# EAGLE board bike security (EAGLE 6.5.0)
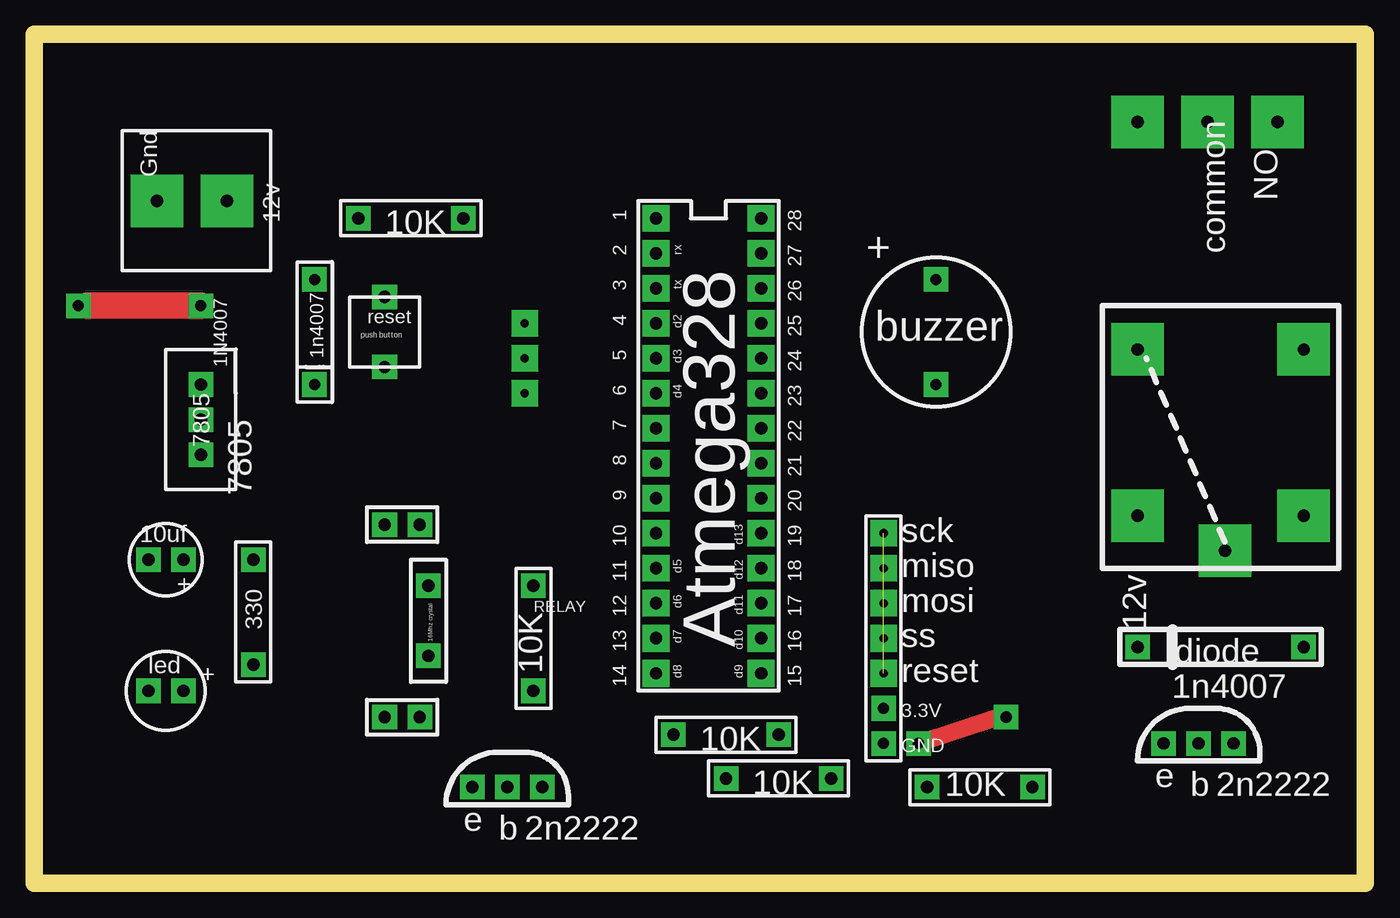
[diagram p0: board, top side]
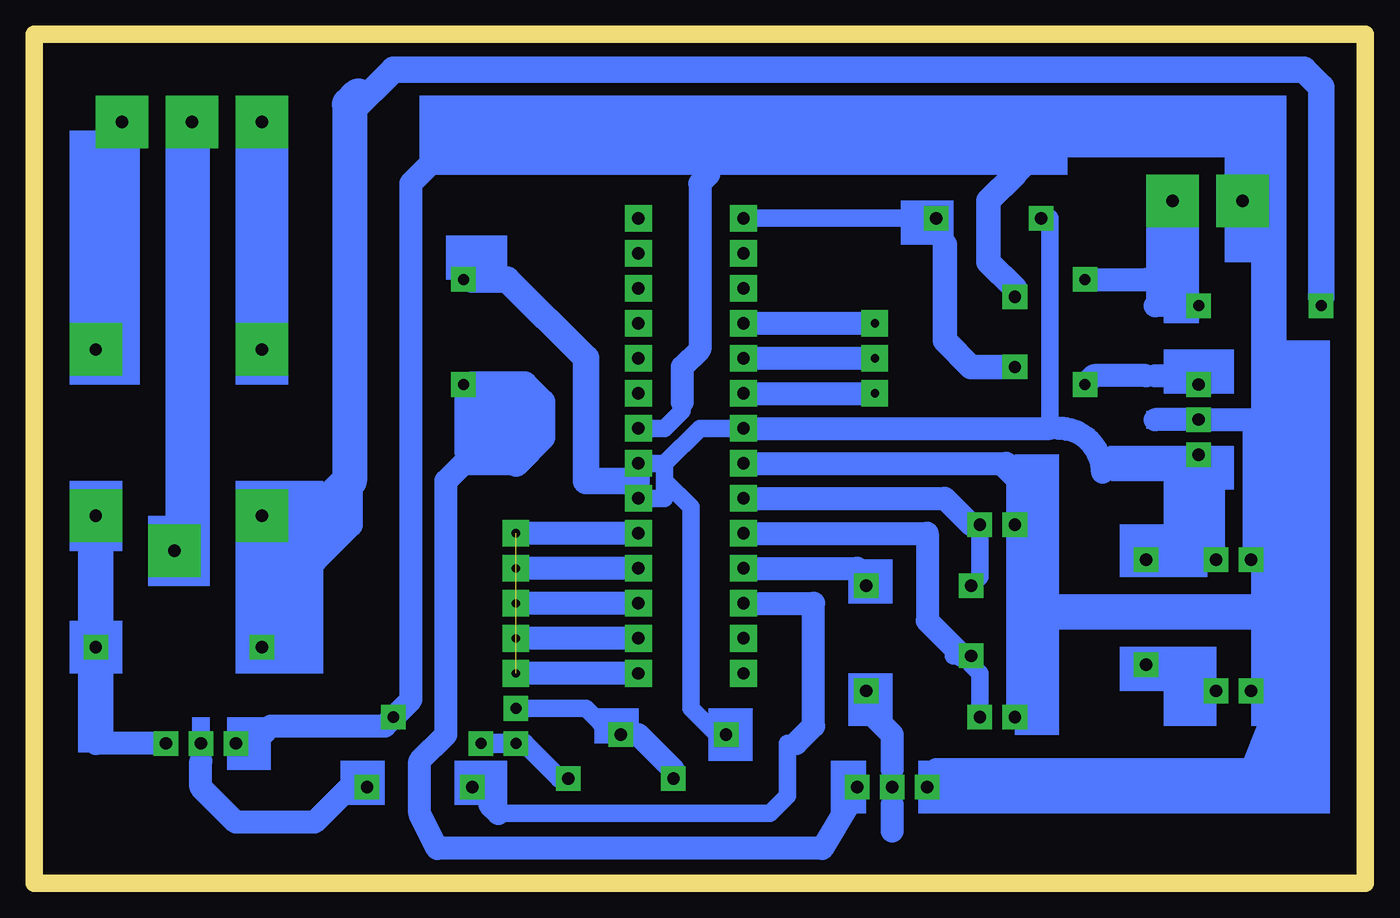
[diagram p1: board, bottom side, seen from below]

Size 96.52 x 61.59 mm. Coordinates in mm from the lower left corner, seen from the top.
Outline: 0,0 96.52,0 96.52,61.59 0,61.59 0,0
Copper layers (1*16): Top 0.035mm / dielectric 1.5mm / Bottom 0.035mm
Design rules "default": minimum track width 10mil, minimum drill 24mil, track to track 8mil, track to pad 8mil, pad to pad 8mil, via to via 8mil, smd to smd 8mil, copper to edge 40mil, drill to drill 8mil, minimum pad ring 10mil, minimum via ring 8mil, stop-mask expansion 4mil, vias tented up to drill 0mil, thermal gap 10mil

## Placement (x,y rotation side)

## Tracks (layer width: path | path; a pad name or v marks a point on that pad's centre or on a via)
S$1
  Bottom 1.27: 29.21,16.51 29.84,16.51 29.84,17.14 31.75,19.05
  Bottom 1.676: 44.45,25.4 31.75,25.4 31.75,19.05 29.21,16.51
S$2  (via drill 0.9 pad 1.93)
  Bottom 1.676: v52.7,27.94 52.7,29.84
  other vias: 52.7,48.26 52.7,45.72 52.7,43.18 52.7,40.64 52.7,38.1 52.7,35.56 52.7,33.02 52.7,30.48 52.7,25.4 52.7,22.86 52.7,20.32 52.7,17.78 45.09,48.26 45.09,45.72 45.09,43.18 45.09,40.64 45.09,38.1 45.09,35.56 45.09,33.02 45.09,30.48 45.09,27.94 45.09,25.4 45.09,22.86 45.09,20.32 45.09,17.78 45.09,15.24
S$3  (via drill 0.8 pad 1.78)
  Bottom 1.676: 80.01,10.79 79.38,11.43 71.12,11.43 v70.48,12.06 69.22,13.34 69.22,50.8 67.31,52.7
S$5  (via drill 0.6 pad 1.93)
  other vias: 35.56,40.64
S$6  (via drill 0.6 pad 1.93)
  other vias: 35.56,38.1
S$7  (via drill 0.9 pad 1.93)
  Bottom 1.27: v52.7,15.24 53.34,15.24
  Bottom 1.676: v52.7,15.24 60.96,15.24 | 52.7,17.78 60.96,17.78 | 52.7,20.32 60.96,20.32 | 52.7,22.86 60.96,22.86 | 52.7,25.4 60.96,25.4
S$8  (via drill 0.6 pad 1.93)
  other vias: 35.56,35.56
S$9  (via drill 0.9 pad 1.78)
  other vias: 80.01,38.73
S$10  (via drill 0.9 pad 1.78)
  other vias: 80.01,26.67
S$11  (via drill 0.9 pad 1.78)
  other vias: 80.01,26.67
S$12  (via drill 0.6 pad 1.93)  (4 unrouted)
  other vias: 61.59,15.24 61.59,17.78 61.59,20.32 61.59,22.86 61.59,25.4
S$13
  Bottom 1.676: 44.45,40.64 36.2,40.64
S$14
  Bottom 1.676: 44.45,38.1 36.2,38.1
S$15
  Bottom 1.676: 44.45,35.56 36.2,35.56
S$16  (via drill 0.9 pad 1.78)
  other vias: 92.08,26.67
S$17  (via drill 0.9 pad 1.78)
  other vias: 80.01,38.73
S$19  (via drill 0.9 pad 1.78)
  other vias: 80.01,38.73
S$20  (via drill 0.9 pad 1.78)
  other vias: 92.08,38.73
S$21  (via drill 0.9 pad 1.78)
  other vias: 86.36,24.13
S$22  (via drill 0.9 pad 1.78)
  other vias: 80.01,17.14
S$23  (via drill 0.9 pad 1.78)
  other vias: 92.08,17.14
S$24
  Bottom 0.813: 80.01,20.95 80.01,19.05
  Bottom 1.422: 80.01,18.41 80.01,20.95
S$25
  Bottom 1.422: 92.08,18.41 92.08,24.77 92.71,24.77
S$26
  Bottom 1.27: 85.72,26.67 85.72,53.98
S$27  (via drill 0.9 pad 3.81)
  other vias: 85.09,55.24 80.01,55.24 80.01,38.73 92.08,38.73 80.01,26.67 86.36,24.13 92.08,26.67
S$28  (via drill 0.9 pad 3.81)
  other vias: 90.17,55.24
S$29
  Bottom 1.27: 92.08,40.64 90.81,41.91 90.81,53.98
S$30
  Bottom 1.676: 87.63,10.16 92.08,10.16
S$31
  Bottom 1.676: 73.66,6.99 76.2,4.45 81.92,4.45 84.45,6.99 84.45,8.89
S$32  (via drill 0.9 pad 1.78)
  other vias: 31.75,6.99
S$33  (via drill 0.9 pad 1.78)
  other vias: 34.29,6.99
S$34  (via drill 0.9 pad 1.78)
  other vias: 36.83,6.99
S$35
  Bottom 1.676: 34.29,8.26 34.29,10.79 35.56,12.06 35.56,12.7
S$36
  Bottom 1.676: 34.29,3.81 34.29,5.71
S$37  (via drill 0.9 pad 1.78)
  other vias: 36.2,21.59
S$38  (via drill 0.9 pad 1.78)
  other vias: 36.2,13.97
S$39
  Bottom 1.676: 6.99,11.43 8.26,8.26 31.11,8.26
S$40
  Bottom 1.676: 6.35,12.06 8.26,6.99 31.11,6.99
S$41
  Bottom 1.676: 37.47,5.71 39.37,2.54 67.31,2.54 68.58,5.08 68.58,8.89 66.67,10.79 66.67,29.21 65.41,30.48 61.59,30.48
  Bottom 1.93: 61.59,30.48 59.69,32.38 59.69,34.92 60.96,36.2 64.77,36.2
S$42  (via drill 0.8 pad 1.78)
  Bottom 1.676: v20.32,43.81 15.88,43.81
S$43
  Bottom 1.676: 19.05,29.84 arc-90 22.23,33.02
S$44
  Bottom 1.676: 13.97,41.91 15.24,41.91
S$45
  Bottom 1.676: 15.24,36.83 13.97,36.83
S$46  (via drill 0.8 pad 1.78)
  other vias: 65.41,43.81
S$47
  Bottom 1.93: 53.34,29.21 56.52,29.21 56.52,38.1 62.23,43.81 64.77,43.81
S$48  (via drill 0.8 pad 1.78)
  Top 1.93: v12.06,41.91 3.81,41.91
S$49  (via drill 0.8 pad 1.78)
  other vias: 65.41,36.2
S$50  (via drill 0.8 pad 1.78)
  other vias: 3.17,41.91
S$51
  Bottom 1.93: 3.17,42.55 3.17,57.78 4.45,59.05 70.48,59.05 73.66,55.88 73.66,29.21 73.66,26.04 76.2,23.5 76.83,23.5
  Bottom 2.54: 73.03,57.15 73.66,56.52 73.66,29.21 74.93,27.94 74.93,25.4
S$52  (via drill 0.9 pad 1.78)
  other vias: 46.35,10.79
S$53  (via drill 0.9 pad 1.78)
  other vias: 53.98,10.79
S$54  (via drill 0.9 pad 1.78)
  other vias: 50.16,7.62
S$55  (via drill 0.9 pad 1.78)
  other vias: 57.78,7.62
S$56
  Bottom 1.676: 50.16,8.26 52.7,10.79 53.34,10.79
S$57
  Bottom 1.676: 62.87,5.08 63.5,5.71
S$58
  Bottom 1.27: 41.91,10.16 41.91,6.35 43.18,5.08 62.23,5.08
S$59  (via drill 0.8 pad 1.78)
  other vias: 61.59,12.7
S$60
  Bottom 1.27: 54.61,10.79 56.52,12.7 60.96,12.7
S$61  (via drill 0.8 pad 1.78)
  other vias: 61.59,10.16
S$62  (via drill 0.8 pad 1.78)
  Top 1.27: v64.14,10.16 69.85,12.06
S$63
  Bottom 1.422: 62.23,10.16 63.5,10.16
S$64
  Bottom 1.422: 60.96,10.16 58.42,7.62
S$65
  Bottom 1.676: 12.7,33.66 15.24,33.66
S$66
  Bottom 1.27: 22.86,33.66 22.86,48.26
S$67  (via drill 0.8 pad 1.78)
  Bottom 1.676: 15.88,36.83 19.68,36.83 v20.32,36.2
S$68
  Bottom 1.27: 18.41,31.11 14.61,30.48 13.97,29.84
S$69
  Bottom 1.27: 46.99,52.07 47.62,51.44 | 52.07,33.02 50.8,33.02 49.53,34.29 49.53,34.92
  Bottom 1.676: 47.62,51.44 48.26,50.8 48.26,38.73 49.53,37.47 49.53,34.92
S$123  (via drill 0.9 pad 1.78)
  other vias: 81.92,10.16
S$125  (via drill 0.9 pad 1.78)
  other vias: 84.45,10.16
S$126  (via drill 0.9 pad 1.78)
  other vias: 87,10.16
S$141  (via drill 0.9 pad 1.78)
  other vias: 72.39,6.99
S$142  (via drill 0.9 pad 1.78)
  other vias: 64.77,6.99
S$319
  Bottom 1.27: 45.09,48.26 33.02,48.26
S$358  (via drill 0.9 pad 1.78)
  other vias: 12.06,36.2
S$359  (via drill 0.9 pad 1.78)
  other vias: 12.06,33.66
S$360  (via drill 0.9 pad 1.78)
  other vias: 12.06,31.11
S$361  (via drill 0.9 pad 1.78)
  Bottom 1.27: v10.79,23.5 10.79,29.21
S$362  (via drill 0.9 pad 1.78)
  Bottom 1.27: v8.26,23.5 8.26,33.66 8.89,33.66
  Bottom 1.676: 11.43,33.66 8.26,33.66
S$363  (via drill 0.9 pad 3.81)
  other vias: 13.97,49.53 8.89,49.53
S$365  (via drill 0.9 pad 1.78)
  other vias: 15.88,15.88
S$366  (via drill 0.9 pad 1.78)
  other vias: 15.88,23.5
S$367  (via drill 0.9 pad 1.78)
  other vias: 10.79,13.97
S$368  (via drill 0.9 pad 1.78)
  other vias: 8.26,13.97
S$392  (via drill 0.9 pad 1.78)
  other vias: 25.4,37.47
S$394  (via drill 0.9 pad 1.78)
  other vias: 25.4,42.55
S$395  (via drill 0.9 pad 1.78)
  other vias: 23.5,48.26
S$396  (via drill 0.9 pad 1.78)
  other vias: 31.11,48.26
S$398
  Bottom 1.778: 26.04,37.47 28.57,37.47 30.48,39.37 30.48,46.35
S$399
  Bottom 1.27: 13.97,53.98 22.86,53.98 27.94,53.98 25.4,52.07
  Bottom 1.676: 25.4,51.44 22.86,53.98
  Bottom 1.778: 25.4,43.18 27.3,45.09 27.3,49.53 25.4,51.44
S$401  (via drill 0.9 pad 1.78)
  Bottom 1.27: v28.57,21.59 27.94,22.23 27.94,25.4
S$402  (via drill 0.9 pad 1.78)
  other vias: 28.57,16.51
S$403  (via drill 0.9 pad 1.78)
  other vias: 25.4,26.04
S$404  (via drill 0.9 pad 1.78)
  other vias: 27.94,26.04
S$405  (via drill 0.9 pad 1.78)
  other vias: 25.4,12.06
S$406  (via drill 0.9 pad 1.78)
  other vias: 27.94,12.06
S$407
  Bottom 1.27: 28.57,15.88 27.94,15.24 27.94,12.7
S$408
  Bottom 1.676: 44.45,27.94 30.48,27.94 28.57,26.04
S$409
  Bottom 1.27: 45.72,33.02 48.26,33.02 50.8,30.48 | 50.8,30.48 52.07,30.48 | 50.8,30.48 50.8,29.21 | 50.8,29.21 50.8,27.94 52.07,27.94 | 50.8,29.21 48.9,27.3 48.9,12.7 46.99,10.79
S$411
  Bottom 1.27: 25.4,25.4 25.4,19.05 | 25.4,19.05 25.4,12.7 | 25.4,19.05 7.62,19.05
S$412
  Bottom 1.676: 44.45,33.02 22.86,33.02
S$413
  Bottom 1.27: 44.45,30.48 26.67,30.48 25.4,29.21 25.4,26.67
  Bottom 1.676: 44.45,30.48 26.04,30.48
S$415
  Bottom 1.27: 44.45,22.86 41.27,22.86
  Bottom 1.676: 44.45,22.86 36.83,22.86
S$416
  Bottom 0.813: 44.45,20.32 41.91,20.32
  Bottom 1.676: 44.45,20.32 40.01,20.32 40.01,11.43 41.27,10.16
(copper drawn outside any net)
  shapes: Bottom area x64

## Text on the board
tPlace: Gnd | 12v | NO | 10K | 1 | 28 | 2 | rx | 27 | common | + | 3 | tx | 26 | reset | 4 | d2 | 25 | push button | 5 | d3 | 24 | buzzer | 1n4007 | 1N4007 | 7805 | 6 | d4 | 23 | 7805 | 7 | 22 | 8 | 21 | 9 | 20 | 10 | d13 | 19 | 10uf | sck | 11 | d5 | d12 | 18 | + | miso | 12 | d6 | d11 | 17 | 16Mhz crystal | RELAY | mosi | 330 | 13 | d7 | d10 | 16 | 12v | diode | Atmega328 | ss | 14 | d8 | d9 | 15 | led | + | 10K | reset | 1n4007 | 3.3V | 10K | GND | 10K | e | 10K | b | 2n2222 | e | b | 2n2222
